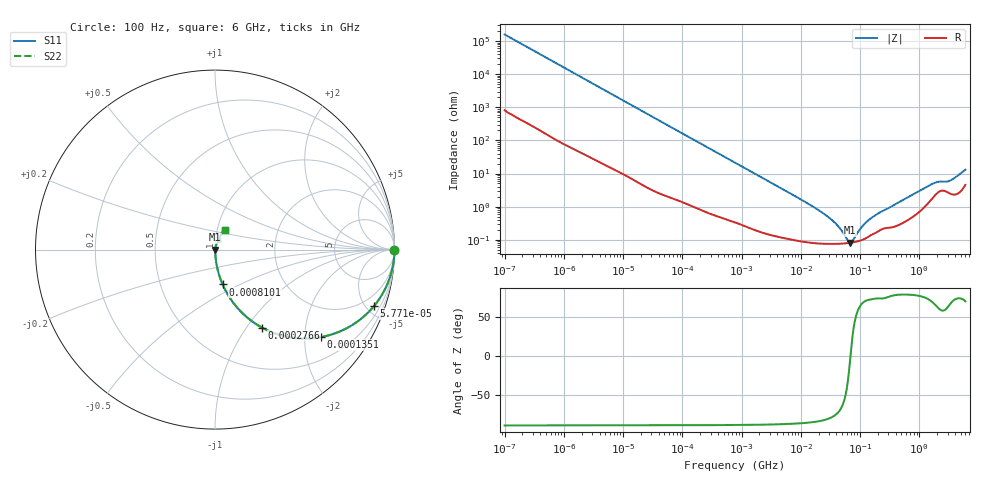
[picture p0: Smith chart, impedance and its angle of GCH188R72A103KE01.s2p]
!Murata Part Number: GCH188R72A103KE01
!These Parameters are Measured in Series Mode Connection
!Data Generated on Mar 13, 2026
!  o--ll--o
!Port1  Port2
!  o------o
!Operation Temp=25[degC], DC Bias Voltage=0[V]
!Freq. Start=100[Hz] Stop=6[GHz] 401[Steps]
# Hz S RI R 50
!Freq.(Hz) S11(Real) S11(Imag) S21(Real) S21(Imag) S12(Real) S12(Imag) S22(Real) S22(Imag)
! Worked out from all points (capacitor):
!   401 points, 100 Hz to 6 GHz, reference 50 ohm
!   read as one part in series: C = 10 nF near 109 Hz
!   lowest |Z| = 81 mohm at 68.17 MHz (marker M1)
!   series resonance near 69.03 MHz, so ESL is about 530 pH
!   S11 on the Smith chart (normalised r, x): 100 Hz: open; 57.71 kHz: 1.04, -5.62; 135.1 kHz: 1.02, -2.41; 276.6 kHz: 1.01, -1.18; 810.1 kHz: 1.01, -0.41; 6 GHz: 1.09, +0.24
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100  1 -0.000629  3.6e-06 0.000629  3.6e-06 0.000629  1 -0.000629
2008  0.9998 -0.0125  0.000222 0.0125  0.000222 0.0125  0.9998 -0.0125
12041  0.994 -0.0741  0.00597 0.0741  0.00597 0.0741  0.994 -0.0741
40335  0.9404 -0.2337  0.0596 0.2337  0.0596 0.2337  0.9404 -0.2337
57709  0.886 -0.3143  0.114 0.3143  0.114 0.3143  0.886 -0.3143
135116  0.5918 -0.487  0.4082 0.487  0.4082 0.487  0.5918 -0.487
276587  0.2614 -0.4341  0.7386 0.4341  0.7386 0.4341  0.2614 -0.4341
452617  0.1193 -0.3177  0.8807 0.3177  0.8807 0.3177  0.1193 -0.3177
774597  0.0462 -0.2022  0.9538 0.2022  0.9538 0.2022  0.0462 -0.2022
810067  0.0426 -0.1942  0.9574 0.1942  0.9574 0.1942  0.0426 -0.1942
2594782  0.00558 -0.0636  0.9944 0.0636  0.9944 0.0636  0.00558 -0.0636
1.555665e7  0.000905 -0.0103  0.9991 0.0103  0.9991 0.0103  0.000905 -0.0103
3.64232e7  0.000759 -0.00336  0.9992 0.00336  0.9992 0.00336  0.000759 -0.00336
6.233367e7  0.000791 -0.000502  0.9992 0.000502  0.9992 0.000502  0.000791 -0.000502
6.817316e7  0.000807 -6.06e-05  0.9992 6.06e-05  0.9992 6.06e-05  0.000807 -6.06e-05
7.455971e7  0.000827 0.00038  0.9992 -0.00038  0.9992 -0.00038  0.000827 0.00038
1.020051e8  0.00095 0.00197  0.999 -0.00197  0.999 -0.00197  0.00095 0.00197
1.334425e8  0.00119 0.00347  0.9988 -0.00347  0.9988 -0.00347  0.00119 0.00347
3.124326e8  0.00238 0.00899  0.9976 -0.00899  0.9976 -0.00899  0.00238 0.00899
1.565993e9  0.0173 0.0421  0.9827 -0.0421  0.9827 -0.0421  0.0173 0.0421
3.205649e9  0.0275 0.0512  0.9725 -0.0512  0.9725 -0.0512  0.0275 0.0512
6e9  0.0563 0.1104  0.9437 -0.1104  0.9437 -0.1104  0.0563 0.1104
